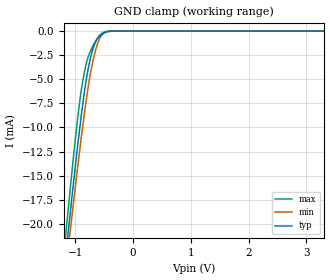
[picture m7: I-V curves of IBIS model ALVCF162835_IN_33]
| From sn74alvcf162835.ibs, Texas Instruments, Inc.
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[Model]   ALVCF162835_IN_33
Model_type  Input
Vinl=0.8
Vinh=2.0
| variable   typ   min   max
C_comp   1.70pF   1.41pF   2.04pF
[Temperature Range]   40   100   -40
| Ambient temperature   25   85   -40
[Voltage range]   3.3   3   3.6
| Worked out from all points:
|   GND clamp passes 1 mA (typ) near -0.64 V on its own axis
[GND Clamp]
| ALVCF162835_IN_33
|   Voltage   I(typ)   I(min)   I(max)
-3.3V     -156.6mA   -149.5mA   -164.8mA
-1.18V    -24.06mA   -25.61mA   -21.95mA
-1.155V   -22.62mA   -24.26mA   -20.4mA
-1.13V    -21.2mA    -22.92mA   -18.86mA
-1.085V   -18.66mA   -20.54mA   -16.12mA
-935mV    -10.6mA    -12.87mA   -7.775mA
-835mV    -5.968mA   -8.175mA   -4.011mA
-755mV    -3.252mA   -4.949mA   -2.301mA
-675mV    -1.496mA   -2.543mA   -1.301mA
-590mV    -591uA     -918.1uA   -519uA
-515mV    -216.8uA   -255.1uA   -135.9uA
3.3V      132.2pA    540.6pA    36.28pA
